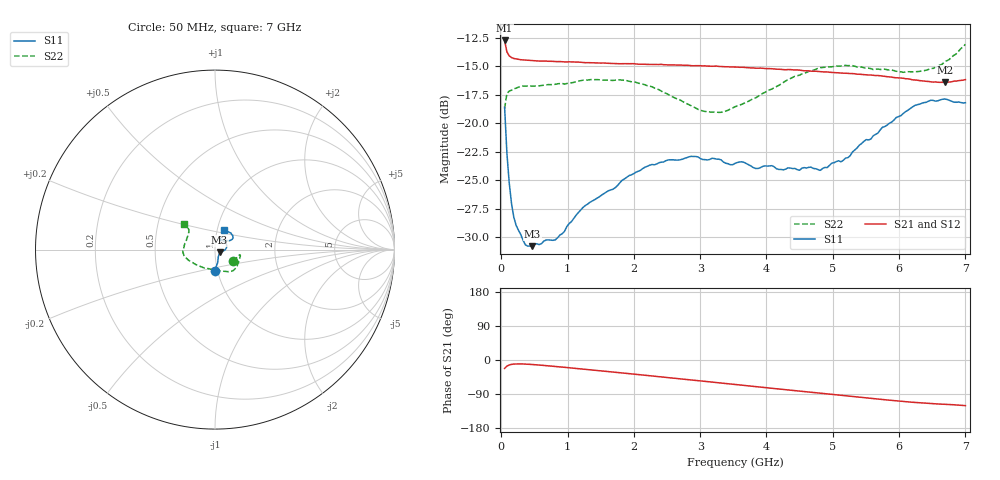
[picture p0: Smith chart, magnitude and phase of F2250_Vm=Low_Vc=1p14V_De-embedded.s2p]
! Integrated Device Technology
! Corporate Headquarters
! 6024 Silver Creek Valley Road
! San Jose, CA 95138  USA
! Phone:  1-408-284-8200
! Toll Free:  1-800-223-1366
! Webpage:  http://www.idt.com/
! Timing and RF Division
! 515 Groton Road, Suite 102
! Westford, MA 01886-6024
! Device:  F2250
! Description: Voltage Variable RF Attenuator
! Frequency:  50.0 -  6000.00 MHz
! Package:  3x3 mm Thin QFN Plastic Package: 16 pin
! Ports:  2 RF, 3 DC
!  Pin  1  = GND
!  Pin  2  = NC
!  Pin  3  = RF1  = Port 1
!  Pin  4  = NC
!  Pin  5  = GND
!  Pin  6  = GND
!  Pin  7  = GND
!  Pin  8  = GND
!  Pin  9  = NC
!  Pin 10  = RF2  = Port 2
!  Pin 11  = NC
!  Pin 12  = GND
!  Pin 13  = GND
!  Pin 14  = VCNTRL
!  Pin 15  = VDD
!  Pin 16  = VMODE
! Vcntrl:  1.140 Volts
! Vmode:  +0.000 Volts
! Vdd:  +3.30  Volts
! Current:  1.191 mA
! Data:  The device was measured on a the F2250 evaluation board which has
!  individual transmission lines to the RF pins.  Data was collected
!  using a calibrated network analyzer.  The evaluation board was
!  de-embedded using a TRL calibration technique.
!  The reference plane is the edge of the package pin.
! Misc:  SN 10
!  Action Tracker AT0258
! Date Measured:  2014-11-26
! Date:  2015-10-15  MJV
! Note:
!  Integrated Device Technology supplies this data as a sample of measured
!  data at the package pin for this product.  Your particular data for this
!  product may vary.
!  Data was taken at 25 degrees C.
!  Integrated Device Technology reserves the right to change this data at anytime.
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# GHz S dB R 50
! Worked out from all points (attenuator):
!   201 points, 50 MHz to 7 GHz, reference 50 ohm
!   highest |S21| = -12.73 dB at 50 MHz (marker M1); lowest = -16.4 dB at 6.687 GHz (marker M2)
!   lowest |S11| = -30.8 dB at 467 MHz (marker M3), VSWR 1.06, Z = 52.6 - j1.48 ohm
!   |S11| at or under -10 dB: start of sweep to end of sweep
!   |S22| runs from -19.0 to -13.1 dB; largest |S21 - S12| = 0.00066
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0.05  -18.58 -91.1  -12.73 -22.2  -12.73 -22.2  -18.70 -32.2
0.08475  -22.64 -78.3  -13.74 -16.1  -13.73 -16.1  -17.39 -17.0
0.1195  -25.23 -71.4  -14.08 -13.1  -14.08 -13.1  -17.18 -12.9
0.189  -28.26 -57.9  -14.31 -10.8  -14.29 -10.8  -16.98 -11.6
0.36275  -30.69 -34.7  -14.44 -10.8  -14.45 -10.8  -16.74 -13.7
0.467  -30.80 -29.3  -14.50 -11.9  -14.49 -11.9  -16.73 -16.0
0.8145  -30.25 -17.8  -14.58 -17.0  -14.58 -17.0  -16.58 -26.4
1.2315  -27.40 -13.3  -14.67 -24.0  -14.65 -24.0  -16.22 -37.1
1.857  -24.89 0.2  -14.76 -34.8  -14.76 -34.8  -16.23 -49.5
2.37825  -23.47 13.1  -14.84 -43.9  -14.82 -43.9  -17.05 -61.1
2.86475  -22.91 28.6  -14.94 -52.6  -14.95 -52.6  -18.47 -79.7
3.0385  -23.19 34.9  -14.96 -55.8  -14.95 -55.8  -18.92 -89.3
3.3165  -23.22 45.2  -15.02 -60.8  -15.01 -60.9  -19.04 -107.2
3.525  -23.53 50.9  -15.05 -64.6  -15.07 -64.6  -18.56 -120.1
3.83775  -23.98 61.5  -15.16 -70.2  -15.17 -70.2  -17.76 -136.4
4.7065  -23.97 62.8  -15.43 -85.9  -15.42 -85.9  -15.34 -165.8
4.81075  -24.14 58.8  -15.46 -87.8  -15.45 -87.8  -15.11 -167.6
5.1235  -23.39 49.0  -15.59 -93.4  -15.57 -93.4  -14.97 -174.6
5.85325  -20.00 31.0  -15.93 -106.0  -15.93 -106.0  -15.34 168.7
6.2355  -18.44 32.7  -16.20 -111.9  -16.19 -112.0  -15.48 156.0
6.68725  -17.87 45.7  -16.41 -116.9  -16.41 -116.9  -14.61 142.1
7  -18.20 64.7  -16.16 -120.4  -16.19 -120.4  -13.06 140.9
